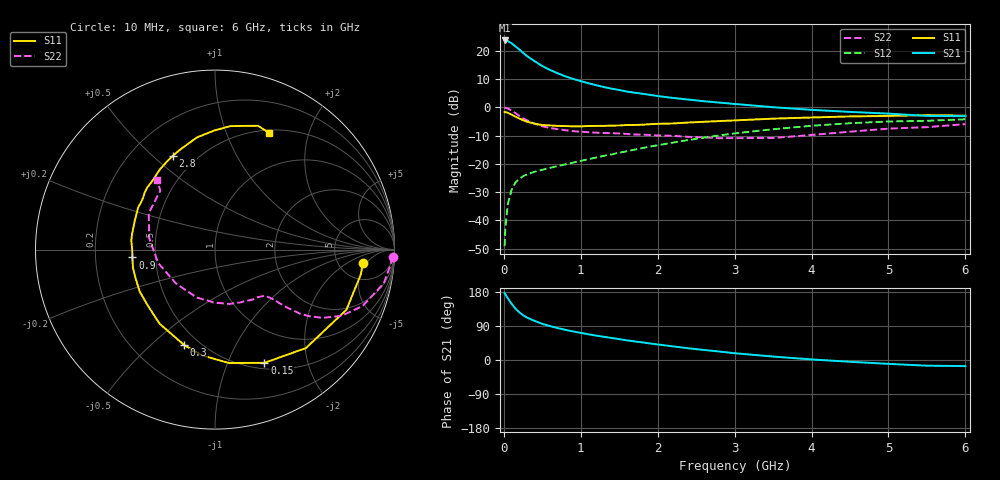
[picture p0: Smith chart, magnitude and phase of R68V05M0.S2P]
! SIEMENS Small Signal Semiconductors
! BFR193
! Si NPN RF Bipolar Junction Transistor in SOT23
! VCE = 8 V  IC = 5 mA
! Common Emitter S-Parameters:  May  1996
# GHz  S  MA  R  50
!  f  S11  S21  S12  S22
! GHz  MAG  ANG  MAG  ANG  MAG  ANG  MAG  ANG
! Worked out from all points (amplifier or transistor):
!   36 points, 10 MHz to 6 GHz, reference 50 ohm
!   highest |S21| = 23.7 dB at 10 MHz (marker M1)
!   |S21| within 3 dB of that: start of sweep to 192.5 MHz
!   unconditionally stable (mu >= 1): 920.6 MHz to 2.022 GHz
!   at 250 MHz: K = 0.42, MSG = 21.8 dB, |S12| = -24.4 dB
!   at 1.4 GHz: K = 1.07, MAG = 10.1 dB, |S12| = -16.6 dB
!   at 6 GHz: K = 0.96, MSG = 0.6 dB, |S12| = -4.2 dB
!   lowest NFmin = 1.20 dB at 450 MHz
!   S11 on the Smith chart (normalised r, x): 10 MHz: 8.65, -4.01; 150 MHz: 0.57, -1.37; 300 MHz: 0.42, -0.64; 900 MHz: 0.37, -0.04; 2.8 GHz: 0.37, +0.58; 6 GHz: 0.54, +1.43
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0.01  0.8266 -5.1  15.32 176.7  0.0035 89.8  0.9901 -2.3
0.02  0.8241 -9.7  15.06 173.1  0.0074 79.4  0.9832 -4.6
0.05  0.8052 -24.6  14.98 163.3  0.0189 77.6  0.959 -11.3
0.1  0.7467 -47.3  13.71 148.6  0.0346 67.3  0.8805 -20.9
0.15  0.6884 -66.4  12.05 135.7  0.0467 59.6  0.7957 -27.6
0.2  0.6368 -83.0  10.65 126.0  0.0542 54.7  0.7119 -32.3
0.25  0.594 -96.8  9.24 118.2  0.0606 51.2  0.6426 -35.3
0.3  0.5593 -107.8  8.129 112.2  0.0653 49.2  0.593 -37.0
0.4  0.5157 -126.6  6.575 103.0  0.0726 47.8  0.5145 -38.8
0.5  0.4873 -140.3  5.406 95.4  0.0789 47.9  0.4625 -39.8
0.6  0.4801 -150.8  4.603 89.5  0.0852 49.1  0.4324 -40.2
0.7  0.4709 -159.8  4.017 84.2  0.0914 50.4  0.4128 -41.0
0.9  0.4622 -174.6  3.201 75.4  0.1055 53.5  0.3805 -42.7
1.1  0.4691 173.8  2.682 67.9  0.1212 56.1  0.3645 -46.0
1.3  0.4713 164.0  2.296 61.2  0.1391 57.8  0.3527 -49.5
1.6  0.4886 151.3  1.909 51.8  0.1674 59.1  0.3393 -56.6
2.2  0.5202 131.2  1.471 35.9  0.2386 57.7  0.3141 -74.7
2.8  0.5728 114.2  1.218 22.4  0.3191 51.8  0.2854 -100.4
3.5  0.6329 99.2  1.009 9.1  0.4113 41.6  0.288 -139.1
4.5  0.6931 83.0  0.833 -4.7  0.5256 25.0  0.3721 170.1
5.5  0.7304 70.8  0.707 -15.0  0.58 7.8  0.4478 132.9
6  0.7161 65.0  0.701 -16.1  0.6169 2.8  0.5061 129.5
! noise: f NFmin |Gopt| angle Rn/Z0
0.45  1.2  0.26  102  0.14
0.9  1.25  0.38  145  0.12
1.8  2.05  0.56  -161  0.12
